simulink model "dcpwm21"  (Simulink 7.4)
settings: Solver=ode45  StartTime=0.0  StopTime=0.7  MaxStep=1e-4  RelTol=1e-3

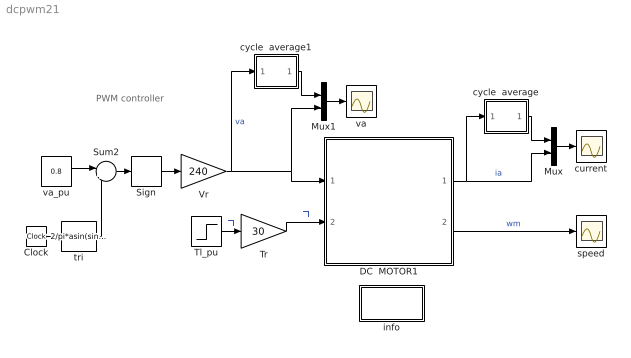
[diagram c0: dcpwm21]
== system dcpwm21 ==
  note: PWM controller
  Clock : Clock
  DC  MOTOR1 : Subsystem  mask{Ra=0.60, La=0.03, J=0.6, Bm=1e-5, K=1.85}
      mask prompts: Ra "Armature resistance [ohm]"; La "Armature inductance [H]"; J "Moment of inertia [Kg.m^2]"; Bm "Frictional torque cefficient"; K "Electromechanical coupling coefficient [N.m/A]"
  Mux : Mux  Inputs=2
  Mux1 : Mux  Inputs=2
  Sign : Signum
  Sum2 : Sum  Inputs=|+-  OutDataType=sfix(16)  OutScaling=2^0
  Tl_pu : Step  Time=0.1  Before=1  After=[.25 .50 0.75 1.0]  SampleTime=0
  Tr : Gain  Gain=30  ParameterDataType=sfix(16)  ParameterScaling=2^0  OutDataType=sfix(16)  OutScaling=2^0
  Vr : Gain  Gain=240  ParameterDataType=sfix(16)  ParameterScaling=2^0  OutDataType=sfix(16)  OutScaling=2^0
  current : Scope
  cycle  average : Subsystem
  cycle  average1 : Subsystem
  info : Subsystem
  speed : Scope
  tri : Fcn  Expr=2/pi*asin(sin(2*pi*1000*u))
  va : Scope
  va_pu : Constant  Value=0.8  OutDataType=sfix(16)  OutScaling=2^0
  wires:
  DC  MOTOR1/2(wm) -> speed/1  "wm"
  cycle  average/1(ave) -> Mux/1
  Mux/1 -> current/1
  DC  MOTOR1/1(ia) -> Mux/2, cycle  average/1(sig)  "ia"
  Sign/1 -> Vr/1
  Tl_pu/1 -> Tr/1  "Tl"
  tri/1 -> Sum2/2
  Sum2/1 -> Sign/1
  Clock/1 -> tri/1
  va_pu/1 -> Sum2/1
  cycle  average1/1(ave) -> Mux1/1
  Mux1/1 -> va/1
  Vr/1 -> cycle  average1/1(sig), DC  MOTOR1/1(va), Mux1/2  "va"
  Tr/1 -> DC  MOTOR1/2(Tl)  "Tl"

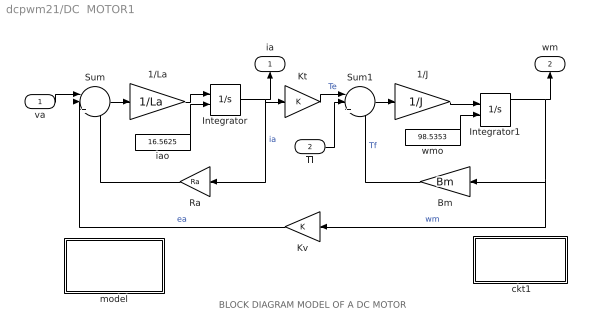
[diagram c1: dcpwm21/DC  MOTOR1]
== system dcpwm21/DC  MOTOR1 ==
  note: BLOCK DIAGRAM MODEL OF A DC MOTOR
  va : Inport  OutDataType=sfix(16)  OutScaling=2^0
  Tl : Inport  Port=2  OutDataType=sfix(16)  OutScaling=2^0
  " ckt1" : Subsystem
  1/J : Gain  Gain=1/J  ParameterDataType=sfix(16)  ParameterScaling=2^0  OutDataType=sfix(16)  OutScaling=2^0
  1/La : Gain  Gain=1/La  ParameterDataType=sfix(16)  ParameterScaling=2^0  OutDataType=sfix(16)  OutScaling=2^0
  Bm : Gain  Gain=Bm  ParameterDataType=sfix(16)  ParameterScaling=2^0  OutDataType=sfix(16)  OutScaling=2^0
  Integrator : Integrator  InitialConditionSource=external  InitialCondition=16.2162
  Integrator1 : Integrator  InitialConditionSource=external  InitialCondition=98.5245
  Kt : Gain  Gain=K  ParameterDataType=sfix(16)  ParameterScaling=2^0  OutDataType=sfix(16)  OutScaling=2^0
  Kv : Gain  Gain=K  ParameterDataType=sfix(16)  ParameterScaling=2^0  OutDataType=sfix(16)  OutScaling=2^0
  Ra : Gain  Gain=Ra  ParameterDataType=sfix(16)  ParameterScaling=2^0  OutDataType=sfix(16)  OutScaling=2^0
  Sum : Sum  Inputs=||+--  OutDataType=sfix(16)  OutScaling=2^0
  Sum1 : Sum  Inputs=||+--  OutDataType=sfix(16)  OutScaling=2^0
  iao : Constant  Value=16.5625  OutDataType=sfix(16)  OutScaling=2^0
  model : Subsystem
  wmo : Constant  Value=98.5353  OutDataType=sfix(16)  OutScaling=2^0
  ia : Outport
  wm : Outport  Port=2
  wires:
  Kv/1 -> Sum/2  "ea"
  Ra/1 -> Sum/3
  Kt/1 -> Sum1/1  "Te"
  Bm/1 -> Sum1/3  "Tf"
  Sum/1 -> 1/La/1
  1/La/1 -> Integrator/1
  Integrator/1 -> Ra/1, Kt/1, ia/1  "ia"
  Sum1/1 -> 1/J/1
  1/J/1 -> Integrator1/1
  Integrator1/1 -> Bm/1, Kv/1, wm/1  "wm"
  va/1 -> Sum/1
  Tl/1 -> Sum1/2
  iao/1 -> Integrator/2
  wmo/1 -> Integrator1/2

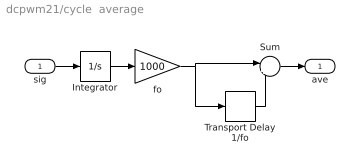
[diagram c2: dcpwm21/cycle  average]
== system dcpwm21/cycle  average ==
  sig : Inport  OutDataType=sfix(16)  OutScaling=2^0
  Integrator : Integrator
  Sum : Sum  Inputs=|+-  OutDataType=sfix(16)  OutScaling=2^0
  Transport Delay 1/fo : TransportDelay  DelayTime=1/1000
  fo : Gain  Gain=1000  ParameterDataType=sfix(16)  ParameterScaling=2^0  OutDataType=sfix(16)  OutScaling=2^0
  ave : Outport
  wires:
  Integrator/1 -> fo/1
  fo/1 -> Sum/1, Transport Delay 1/fo/1
  sig/1 -> Integrator/1
  Transport Delay 1/fo/1 -> Sum/2
  Sum/1 -> ave/1

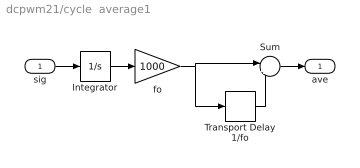
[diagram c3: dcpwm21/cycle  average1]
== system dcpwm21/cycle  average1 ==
  sig : Inport  OutDataType=sfix(16)  OutScaling=2^0
  Integrator : Integrator
  Sum : Sum  Inputs=|+-  OutDataType=sfix(16)  OutScaling=2^0
  Transport Delay 1/fo : TransportDelay  DelayTime=1/1000
  fo : Gain  Gain=1000  ParameterDataType=sfix(16)  ParameterScaling=2^0  OutDataType=sfix(16)  OutScaling=2^0
  ave : Outport
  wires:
  Integrator/1 -> fo/1
  fo/1 -> Sum/1, Transport Delay 1/fo/1
  sig/1 -> Integrator/1
  Transport Delay 1/fo/1 -> Sum/2
  Sum/1 -> ave/1

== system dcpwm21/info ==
  note: This demo simulates the running of a DC motor with PWM (bipolar) excitation (5 hp 240V 1200 rpm) rated torque Tr = 30 N.m

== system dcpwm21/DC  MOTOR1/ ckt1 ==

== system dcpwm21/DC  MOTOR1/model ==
  note: Electrical system equation: va = Ra.ia + La.dia/dt + ea where ea = K.wm Mechanical system equation: Te = J.dwm/dt + Tl.signum(wm) + f(wm) where Te = K.ia
  note: Mathematical model of the dc machine
